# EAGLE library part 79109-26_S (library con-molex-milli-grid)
RECEPTACAL
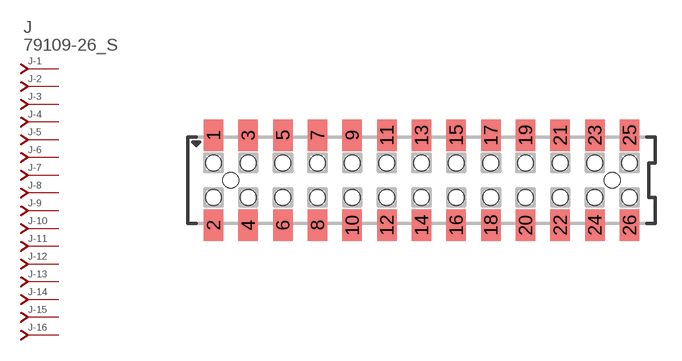
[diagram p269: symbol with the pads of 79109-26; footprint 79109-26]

Designator prefix J; gates -1=J-NV -2=J-N -3=J-N -4=J-N -5=J-N -6=J-N -7=J-N -8=J-N -9=J-N -10=J-N -11=J-N -12=J-N -13=J-N -14=J-N -15=J-N -16=J-N -17=J-N -18=J-N -19=J-N -20=J-N -21=J-N -22=J-N -23=J-N -24=J-N -25=J-N -26=J-N

## 79109-26_S  [79109-26]
1  -1:J  pas
2  -2:J  pas
3  -3:J  pas
4  -4:J  pas
5  -5:J  pas
6  -6:J  pas
7  -7:J  pas
8  -8:J  pas
9  -9:J  pas
10  -10:J  pas
11  -11:J  pas
12  -12:J  pas
13  -13:J  pas
14  -14:J  pas
15  -15:J  pas
16  -16:J  pas
17  -17:J  pas
18  -18:J  pas
19  -19:J  pas
20  -20:J  pas
21  -21:J  pas
22  -22:J  pas
23  -23:J  pas
24  -24:J  pas
25  -25:J  pas
26  -26:J  pas

## Footprint 79109-26 (pad centres in mm)
RECEPTACAL SMD Dual Row, Vertical, Pass-Thru
smd 1.12 x 1.83: 1 -12,2.6; 2 -12,-2.6; 3 -10,2.6; 4 -10,-2.6; 5 -8,2.6; 6 -8,-2.6; 7 -6,2.6; 8 -6,-2.6; 9 -4,2.6; 10 -4,-2.6; 11 -2,2.6; 12 -2,-2.6; 13 0,2.6; 14 0,-2.6; 15 2,2.6; 16 2,-2.6; 17 4,2.6; 18 4,-2.6; 19 6,2.6; 20 6,-2.6; 21 8,2.6; 22 8,-2.6; 23 10,2.6; 24 10,-2.6; 25 12,2.6; 26 12,-2.6
hole 0.914 at -11,0
hole 0.914 at -12,1
hole 0.914 at -12,-1
hole 0.914 at -10,-1
hole 0.914 at -10,1
hole 0.914 at -8,-1
hole 0.914 at -8,1
hole 0.914 at 11,0
hole 0.914 at -6,1
hole 0.914 at -6,-1
hole 0.914 at -4,1
hole 0.914 at -4,-1
hole 0.914 at -2,1
hole 0.914 at -2,-1
hole 0.914 at 0,1
hole 0.914 at 0,-1
hole 0.914 at 2,-1
hole 0.914 at 2,1
hole 0.914 at 4,1
hole 0.914 at 4,-1
hole 0.914 at 6,1
hole 0.914 at 6,-1
hole 0.914 at 8,1
hole 0.914 at 8,-1
hole 0.914 at 10,-1
hole 0.914 at 10,1
hole 0.914 at 12,1
hole 0.914 at 12,-1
